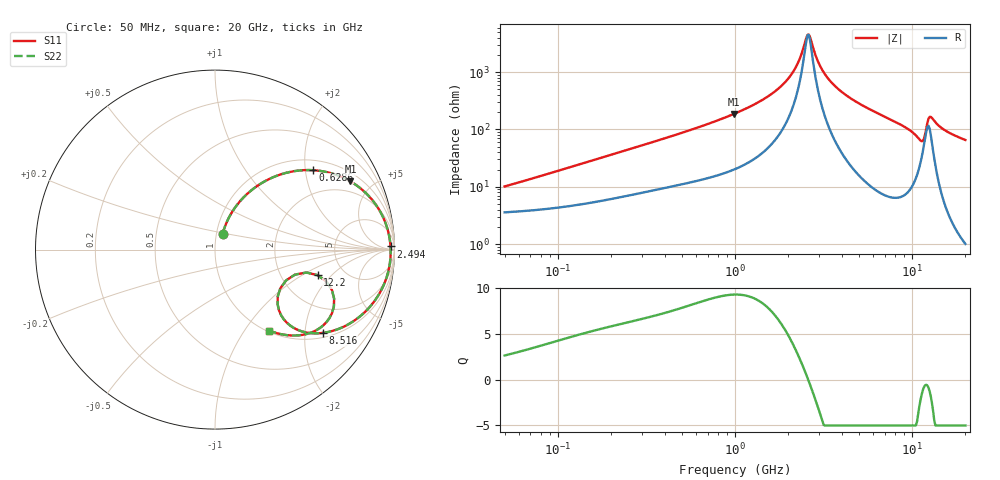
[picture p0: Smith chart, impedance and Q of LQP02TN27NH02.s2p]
!Murata Part Number: LQP02TN27NH02
!These Parameters are Measured in Series Mode Connection
!  o--[Z]--o
!Port1  Port2
!  o-------o
!Freq. Start=50[MHz] Stop=20[GHz], 401[Steps]
# Hz S RI R 50
!Freq.(Hz) S11(Real) S11(Imag) S21(Real) S21(Imag) S12(Real) S12(Imag) S22(Real) S22(Imag)
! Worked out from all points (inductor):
!   401 points, 50 MHz to 20 GHz, reference 50 ohm
!   read as one part in series: L = 29.7 nH near 58.96 MHz
!   highest Q = 9.32 at 985.1 MHz (marker M1), where L = 30 nH
!   self-resonance near 2.569 GHz
!   S11 on the Smith chart (normalised r, x): 50 MHz: 1.07, +0.19; 628.6 MHz: 1.26, +2.20; 2.494 GHz: 54, +44; 8.516 GHz: 1.13, -2.48; 12.2 GHz: 3.20, -1.40; 20 GHz: 1.02, -1.31
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5e7  0.0425 0.0876  0.9575 -0.0876  0.9575 -0.0876  0.0425 0.0876
1.364002e8  0.0976 0.2135  0.9024 -0.2135  0.9024 -0.2135  0.0976 0.2135
3.721004e8  0.321 0.402  0.679 -0.402  0.679 -0.402  0.321 0.402
6.285508e8  0.5448 0.4425  0.4552 -0.4425  0.4552 -0.4425  0.5448 0.4425
9.85133e8  0.7545 0.38  0.2455 -0.38  0.2455 -0.38  0.7545 0.38
1e9  0.7609 0.3762  0.2391 -0.3762  0.2391 -0.3762  0.7609 0.3762
1.432596e9  0.8904 0.2582  0.1096 -0.2582  0.1096 -0.2582  0.8904 0.2582
1.875929e9  0.9508 0.1463  0.0492 -0.1463  0.0492 -0.1463  0.9508 0.1463
2.211938e9  0.9711 0.0727  0.0289 -0.0727  0.0289 -0.0727  0.9711 0.0727
2.493527e9  0.9779 0.0177  0.0221 -0.0177  0.0221 -0.0177  0.9779 0.0177
2.608132e9  0.9788 -0.00307  0.0212 0.00307  0.0212 0.00307  0.9788 -0.00307
2.728004e9  0.9787 -0.0239  0.0213 0.0239  0.0213 0.0239  0.9787 -0.0239
3.075291e9  0.9738 -0.0798  0.0262 0.0798  0.0262 0.0798  0.9738 -0.0798
3.736399e9  0.9507 -0.1704  0.0493 0.1704  0.0493 0.1704  0.9507 -0.1704
7.442007e9  0.6926 -0.4402  0.3074 0.4402  0.3074 0.4402  0.6926 -0.4402
8.516016e9  0.6006 -0.4641  0.3994 0.4641  0.3994 0.4641  0.6006 -0.4641
1.004137e10  0.4511 -0.4427  0.5489 0.4427  0.5489 0.4427  0.4511 -0.4427
1.115139e10  0.3486 -0.3027  0.6514 0.3027  0.6514 0.3027  0.3486 -0.3027
1.220001e10  0.5715 -0.1423  0.4285 0.1423  0.4285 0.1423  0.5715 -0.1423
1.295331e10  0.6624 -0.3165  0.3376 0.3165  0.3376 0.3165  0.6624 -0.3165
1.438523e10  0.5494 -0.4567  0.4506 0.4567  0.4506 0.4567  0.5494 -0.4567
2e10  0.3027 -0.4518  0.6973 0.4518  0.6973 0.4518  0.3027 -0.4518
